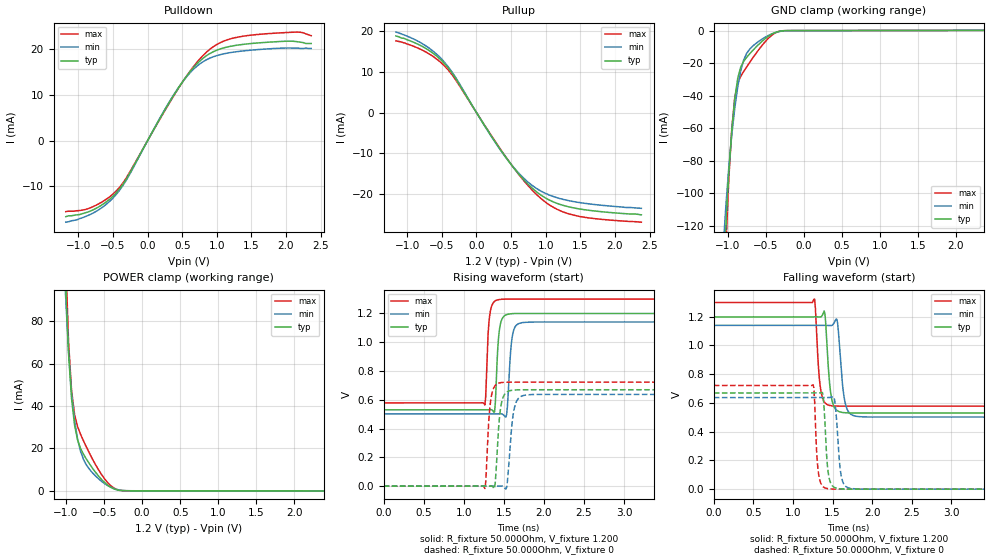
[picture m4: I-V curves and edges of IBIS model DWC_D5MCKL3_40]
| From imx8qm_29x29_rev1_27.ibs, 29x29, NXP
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[Model] DWC_D5MCKL3_40
Model_type   I/O
Polarity   Non-Inverting
Enable   Active-High
C_comp   1.264pF   1.181pF   1.367pF
C_comp_pullup   284.432fF   261.981fF   311.497fF
C_comp_pulldown 969.059fF   903.013fF   1.049pF
Vinh = 975.000mV
Vinl = 705.000mV
Vmeas = 840.000mV
Vref = 840.000mV
Rref = 50Ohms
Cref = 5pF
[Model Spec]
Vinh   975.000mV   933.000mV   1.045V
Vinl   705.000mV   663.000mV   775.000mV
Vmeas   840.000mV   798.000mV   910.000mV
Vref   840.000mV   798.000mV   910.000mV
D_overshoot_ampl_h 0.35 NA   NA
D_overshoot_ampl_l 0.35 NA   NA
D_overshoot_area_l 100.000p NA   NA
D_overshoot_area_h 100.000p NA   NA
[Receiver Thresholds]
Vcross_low = 720.000mV
Vcross_high = 960.000mV
Vdiff_ac = 270.000mV
Vdiff_dc = 200.000mV
Tdiffslew_ac = 10.000ns
[Temperature Range]   25.000   125.000   -40.000
[Voltage Range]   1.200V   1.140V   1.300V
[GND Clamp Reference]   0.00V   0.00V   0.00V
[C Comp Corner]
| variable   typ   min   max
C_comp 1.264pF   1.367pF   1.181pF
C_comp_pullup 284.432fF   311.497fF   261.981fF
C_comp_pulldown 969.059fF   1.049pF   903.013fF
[Pulldown Reference]   0.00V   0.00V   0.00V
[POWER Clamp Reference]   1.200V   1.140V   1.300V
[Pullup Reference]   1.200V   1.140V   1.300V
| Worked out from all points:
|   slope of the pulldown table from 0 to 0.18 V, typ, clamps not added: 37.1 ohm
|   slope of the pullup table from 0 to 0.18 V, typ, clamps not added: 37.2 ohm
|   GND clamp passes 1 mA (typ) near -0.36 V on its own axis
|   POWER clamp passes 1 mA (typ) near -0.38 V on its own axis
|   rising waveform, R_fixture 50.000Ohm, V_fixture 1.200: 20-80 % time 39.8ps typ, 45.6ps min, 37.3ps max; typ from 0.53 V to 1.2 V
|   rising waveform, R_fixture 50.000Ohm, V_fixture 0: 20-80 % time 52.2ps typ, 61.3ps min, 47.1ps max; typ from 0 V to 0.669 V
|   falling waveform, R_fixture 50.000Ohm, V_fixture 1.200: 20-80 % time 55.4ps typ, 63.8ps min, 50ps max; typ from 1.2 V to 0.53 V
|   falling waveform, R_fixture 50.000Ohm, V_fixture 0: 20-80 % time 44.8ps typ, 53.2ps min, 38.9ps max; typ from 0.669 V to 0 V
[GND Clamp]
-1.182V   -339.3mA   -254.8mA   -426.6mA
-1.064V   -163.5mA   -137.8mA   -190.4mA
-1.024V   -121.1mA   -108.6mA   -134.3mA
-984.8mV  -87.5mA    -84.22mA   -91.46mA
-945.5mV  -61.36mA   -64.12mA   -60.5mA
-906.1mV  -41.91mA   -47.62mA   -41.1mA
-866.7mV  -29.17mA   -34.43mA   -32.17mA
-827.3mV  -22.35mA   -24.56mA   -28.07mA
-748.5mV  -16.34mA   -13.87mA   -22.22mA
-590.9mV  -8.454mA   -6.602mA   -11.71mA
-275.8mV  -116.4uA   -248.8uA   -84.78uA
2.364V    136.6uA    111.3uA    170.2uA
[Power Clamp]
-1.164V   362.5mA    268.1mA    465.2mA
-1.006V   98.99mA    92.43mA    111.8mA
-966.7mV  64.74mA    65.63mA    70.25mA
-927.3mV  43.55mA    46.45mA    47.41mA
-887.9mV  31.08mA    33.31mA    36.05mA
-848.5mV  24.04mA    24.48mA    30.35mA
-809.1mV  19.97mA    18.62mA    26.67mA
-690.9mV  12.66mA    10.09mA    17.63mA
-493.9mV  3.911mA    3.404mA    5.643mA
-375.8mV  976.4uA    1.116mA    1.399mA
-257.6mV  56.8uA     160.4uA    65.6uA
2.382V    -68.29uA   -58.74uA   -77.9uA
[Pulldown]
-1.182V   -16.6mA    -17.8mA    -15.5mA
-827.3mV  -15.38mA   -16.1mA    -14.66mA
-630.3mV  -13.73mA   -14.29mA   -13.12mA
-433.3mV  -11.07mA   -11.38mA   -10.68mA
-275.8mV  -7.56mA    -7.806mA   -7.327mA
354.5mV   9.334mA    9.459mA    9.199mA
551.5mV   13.82mA    13.72mA    13.83mA
748.5mV   17.28mA    16.67mA    17.72mA
984.8mV   19.64mA    18.48mA    20.84mA
1.3V      20.84mA    19.43mA    22.57mA
2.127V    21.65mA    20.18mA    23.67mA
2.364V    21.2mA     20.1mA     22.9mA
[Pullup]
-1.164V   18.8mA     19.75mA    17.61mA
-730.3mV  15.72mA    16.35mA    14.85mA
-572.7mV  13.82mA    14.28mA    13.1mA
-415.1mV  11.07mA    11.37mA    10.58mA
-297mV    8.231mA    8.487mA    7.928mA
372.7mV   -9.747mA   -9.831mA   -9.632mA
609.1mV   -15.06mA   -14.85mA   -15.14mA
806.1mV   -18.57mA   -17.9mA    -19.05mA
1.042V    -21.38mA   -20.17mA   -22.53mA
1.318V    -23.07mA   -21.56mA   -24.77mA
1.673V    -24.08mA   -22.5mA    -25.96mA
2.382V    -25.1mA    -23.5mA    -26.9mA
[Ramp]
R_load=50.000Ohm
dV/dt_r   401.250mV/46.500ps  382.229mV/54.000ps  432.480mV/42.500ps
dV/dt_f   401.280mV/50.500ps  382.229mV/59.000ps  432.510mV/45.500ps
[Rising waveform]
R_fixture=50.000Ohm
V_fixture=1.200
V_fixture_min=1.140
V_fixture_max=1.300
0s        529.9mV    501.6mV    577.8mV
1.263ns   529.9mV    501.6mV    562.9mV
1.323ns   530.7mV    501.6mV    1.185V
1.383ns   515.2mV    501.5mV    1.282V
1.423ns   951mV      502mV      1.293V
1.454ns   1.118V     502.8mV    1.296V
1.534ns   1.19V      496.2mV    1.298V
1.614ns   1.197V     1.065V     1.298V
1.734ns   1.198V     1.135V     1.298V
10ns      1.198V     1.139V     1.298V
[Rising waveform]
R_fixture=50.000Ohm
V_fixture=0
0s        184.5nV    4.611uV    25.69nV
1.263ns   -4.332uV   3.448uV    -16.16mV
1.343ns   1.37mV     7.193uV    622.4mV
1.383ns   -16.68mV   -94.96uV   691.8mV
1.444ns   471.6mV    961.4uV    716.2mV
1.474ns   586.8mV    1.319mV    719.3mV
1.534ns   652mV      -9.097mV   721.3mV
1.634ns   667.3mV    549.7mV    721.8mV
1.774ns   669.1mV    632.3mV    721.9mV
10ns      668.9mV    636.8mV    721.4mV
[Falling waveform]
R_fixture=50.000Ohm
V_fixture=1.200
V_fixture_min=1.140
V_fixture_max=1.300
0s        1.198V     1.139V     1.298V
1.273ns   1.199V     1.139V     1.322V
1.333ns   1.198V     1.139V     768.7mV
1.403ns   1.221V     1.139V     601.4mV
1.484ns   641.5mV    1.138V     580mV
1.564ns   543.9mV    1.151V     577.5mV
1.624ns   533.4mV    733mV      577.2mV
1.664ns   531.3mV    588.5mV    577.2mV
1.814ns   529.6mV    505.6mV    577.2mV
10ns      529.8mV    501.6mV    577.6mV
[Falling waveform]
R_fixture=50.000Ohm
V_fixture=0
0s        668.9mV    636.8mV    721.3mV
1.253ns   668.9mV    636.8mV    726.1mV
1.263ns   668.9mV    636.8mV    706.2mV
1.323ns   668.5mV    636.8mV    105.2mV
1.383ns   635.5mV    636.8mV    15.96mV
1.444ns   117.4mV    636.4mV    3.038mV
1.524ns   11.8mV     623.6mV    385.4uV
1.614ns   1.674mV    78.77mV    41.83uV
1.744ns   123.5uV    4.112mV    7.594uV
10ns      429.2nV    4.823uV    94.92nV
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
